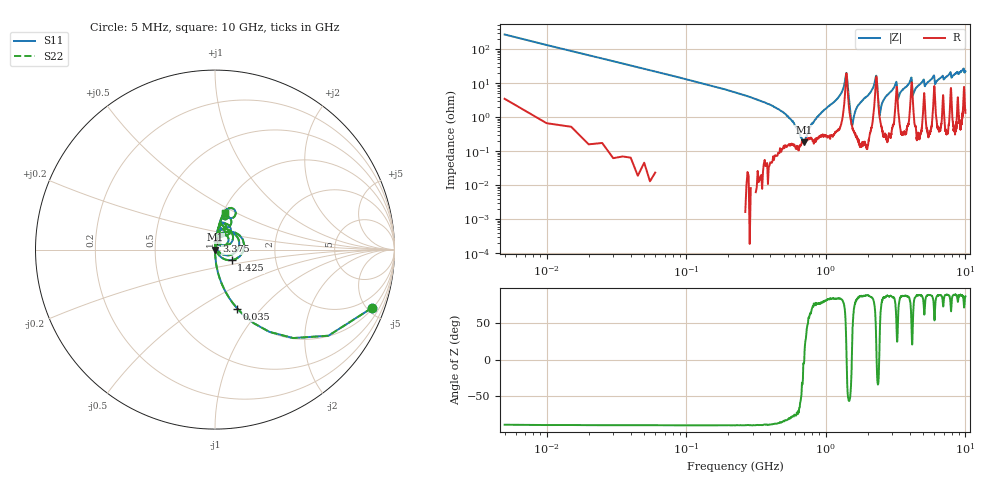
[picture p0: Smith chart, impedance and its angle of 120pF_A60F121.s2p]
! Amotech Co.,Ltd.
! http://www.amotech.co.kr/
! Part Number: A60F121
! These Parameters are Measured in Series Mode Connection
! Operation Temp=25[degC], DC Bias Voltage=0[V]
! Freq. Start=5[MHz] Stop=10[GHz], 2000[Steps]
! Date: Monday, July 20, 2020, 04:45:02
# GHZ S RI R 50.000000
!Freq.(Hz) S11(Real) S11(Imag) S21(Real) S21(Imag) S12(Real) S12(Imag) S22(Real) S22(Imag)
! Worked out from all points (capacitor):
!   2000 points, 5 MHz to 10 GHz, reference 50 ohm
!   read as one part in series: C = 121 pF near 55 MHz
!   lowest |Z| = 183 mohm at 695 MHz (marker M1)
!   series resonance near 701 MHz, so ESL is about 430 pH
!   S11 on the Smith chart (normalised r, x): 5 MHz: 1.07, -5.36; 35 MHz: 1.00, -0.75; 1.425 GHz: 1.19, -0.14; 3.375 GHz: 1.01, +0.09; 10 GHz: 1.03, +0.44
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0.005  0.8745 -0.3249  0.1255 0.3249  0.1255 0.3249  0.8745 -0.3249
0.035  0.124 -0.3287  0.876 0.3287  0.876 0.3287  0.124 -0.3287
0.145  0.00731 -0.0862  0.9927 0.0862  0.9927 0.0862  0.00731 -0.0862
0.49  0.00134 -0.0142  0.9987 0.0142  0.9987 0.0142  0.00134 -0.0142
0.695  0.00181 -0.000183  0.9982 0.000183  0.9982 0.000183  0.00181 -0.000183
0.91  0.00294 0.0118  0.9971 -0.0118  0.9971 -0.0118  0.00294 0.0118
1.375  0.06 0.0968  0.94 -0.0968  0.94 -0.0968  0.06 0.0968
1.425  0.0921 -0.059  0.9079 0.059  0.9079 0.059  0.0921 -0.059
1.54  0.00534 0.001  0.9947 -0.001  0.9947 -0.001  0.00534 0.001
1.675  0.0029 0.0194  0.9971 -0.0194  0.9971 -0.0194  0.0029 0.0194
2.275  0.0911 0.0958  0.9089 -0.0958  0.9089 -0.0958  0.0911 0.0958
2.44  0.00901 0.00752  0.991 -0.00752  0.991 -0.00752  0.00901 0.00752
2.645  0.00424 0.0356  0.9958 -0.0356  0.9958 -0.0356  0.00424 0.0356
3.17  0.0399 0.0872  0.9601 -0.0872  0.9601 -0.0872  0.0399 0.0872
3.34  0.0117 0.0393  0.9883 -0.0393  0.9883 -0.0393  0.0117 0.0393
3.375  0.00868 0.0459  0.9913 -0.0459  0.9913 -0.0459  0.00868 0.0459
4.07  0.0605 0.115  0.9395 -0.115  0.9395 -0.115  0.0605 0.115
4.23  0.0209 0.0403  0.9791 -0.0403  0.9791 -0.0403  0.0209 0.0403
5.005  0.0365 0.1152  0.9635 -0.1152  0.9635 -0.1152  0.0365 0.1152
6.67  0.0253 0.1393  0.9747 -0.1393  0.9747 -0.1393  0.0253 0.1393
8.335  0.0353 0.1728  0.9647 -0.1728  0.9647 -0.1728  0.0353 0.1728
10  0.0581 0.2058  0.9419 -0.2058  0.9419 -0.2058  0.0581 0.2058
